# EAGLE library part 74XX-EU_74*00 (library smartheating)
Quad 2-input NAND gate
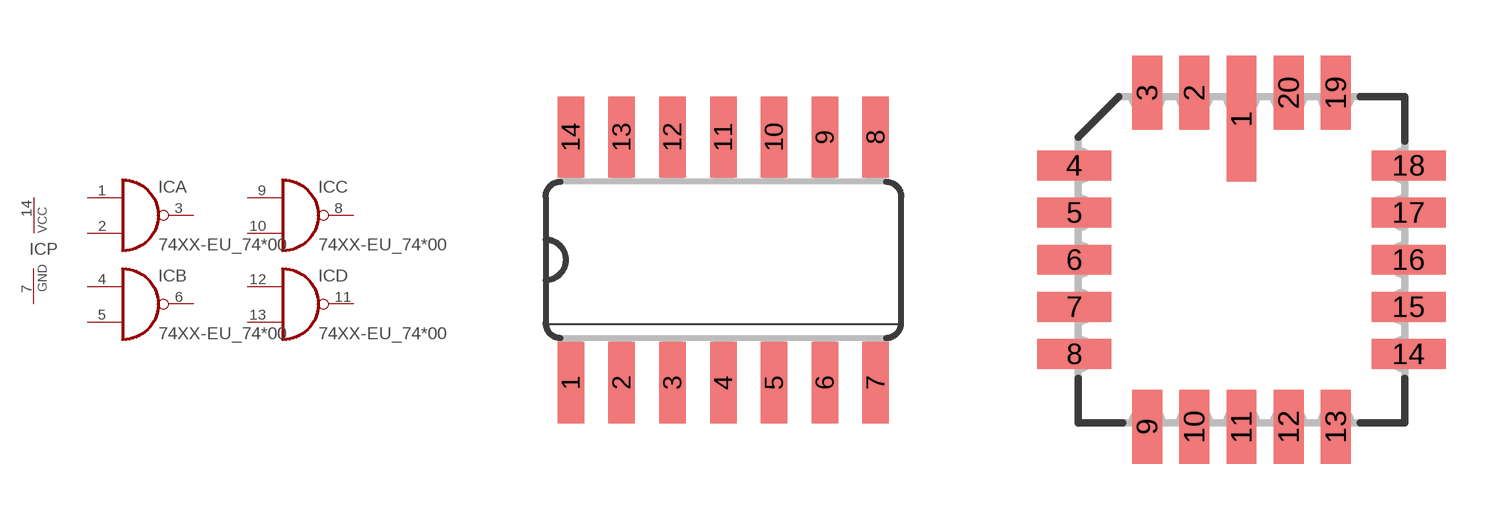
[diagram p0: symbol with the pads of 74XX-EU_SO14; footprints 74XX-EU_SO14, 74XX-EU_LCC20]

Designator prefix IC; gates A=74XX-EU_7400 B=74XX-EU_7400 C=74XX-EU_7400 D=74XX-EU_7400 P=74XX-EU_PWRN

## 74XX-EU_7400D, 74XX-EU_74AC00D, 74XX-EU_74ACT00D, 74XX-EU_74ALS00D, 74XX-EU_74AS00D, 74XX-EU_74HC00D, 74XX-EU_74HCT00D, 74XX-EU_74LS00D, 74XX-EU_74S00D  [74XX-EU_SO14]
1  A:I0  in
2  A:I1  in
3  A:O  out
4  B:I0  in
5  B:I1  in
6  B:O  out
7  P:GND  pwr
8  C:O  out
9  C:I0  in
10  C:I1  in
11  D:O  out
12  D:I0  in
13  D:I1  in
14  P:VCC  pwr

## 74XX-EU_7400FK, 74XX-EU_74AC00FK, 74XX-EU_74ACT00FK, 74XX-EU_74ALS00FK, 74XX-EU_74AS00FK, 74XX-EU_74HC00FK, 74XX-EU_74HCT00FK, 74XX-EU_74LS00FK, 74XX-EU_74S00FK  [74XX-EU_LCC20]
2  A:I0  in
3  A:I1  in
4  A:O  out
6  B:I0  in
8  B:I1  in
9  B:O  out
10  P:GND  pwr
12  C:O  out
13  C:I0  in
14  C:I1  in
16  D:O  out
18  D:I0  in
19  D:I1  in
20  P:VCC  pwr

## 74XX-EU_7400N, 74XX-EU_74AC00N, 74XX-EU_74ACT00N, 74XX-EU_74ALS00N, 74XX-EU_74AS00N, 74XX-EU_74HC00N, 74XX-EU_74HCT00N, 74XX-EU_74LS00N, 74XX-EU_74S00N  [74XX-EU_DIL14]
Pads as for 74XX-EU_SO14

## Footprint 74XX-EU_SO14 (pad centres in mm)
Small Outline package 150 mil
smd 0.66 x 2.032: 1 -3.81,-3.073; 2 -2.54,-3.073; 3 -1.27,-3.073; 4 0,-3.073; 5 1.27,-3.073; 6 2.54,-3.073; 7 3.81,-3.073; 8 3.81,3.073; 9 2.54,3.073; 10 1.27,3.073; 11 0,3.073; 12 -1.27,3.073; 13 -2.54,3.073; 14 -3.81,3.073

## Footprint 74XX-EU_LCC20 (pad centres in mm)
Leadless Chip Carrier Ceramic Package
smd 0.8 x 3.4: 1 0,3.8
smd 0.8 x 2: 2 -1.27,4.5; 3 -2.54,4.5; 9 -2.54,-4.5; 10 -1.27,-4.5; 11 0,-4.5; 12 1.27,-4.5; 13 2.54,-4.5; 19 2.54,4.5; 20 1.27,4.5
smd 2 x 0.8: 4 -4.5,2.54; 5 -4.5,1.27; 6 -4.5,0; 7 -4.5,-1.27; 8 -4.5,-2.54; 14 4.5,-2.54; 15 4.5,-1.27; 16 4.5,0; 17 4.5,1.27; 18 4.5,2.54

## Footprint 74XX-EU_DIL14 (pad centres in mm)
Dual In Line Package
drill 0.813 long: 1 -7.62,-3.81; 2 -5.08,-3.81; 3 -2.54,-3.81; 4 0,-3.81; 5 2.54,-3.81; 6 5.08,-3.81; 7 7.62,-3.81; 8 7.62,3.81; 9 5.08,3.81; 10 2.54,3.81; 11 0,3.81; 12 -2.54,3.81; 13 -5.08,3.81; 14 -7.62,3.81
